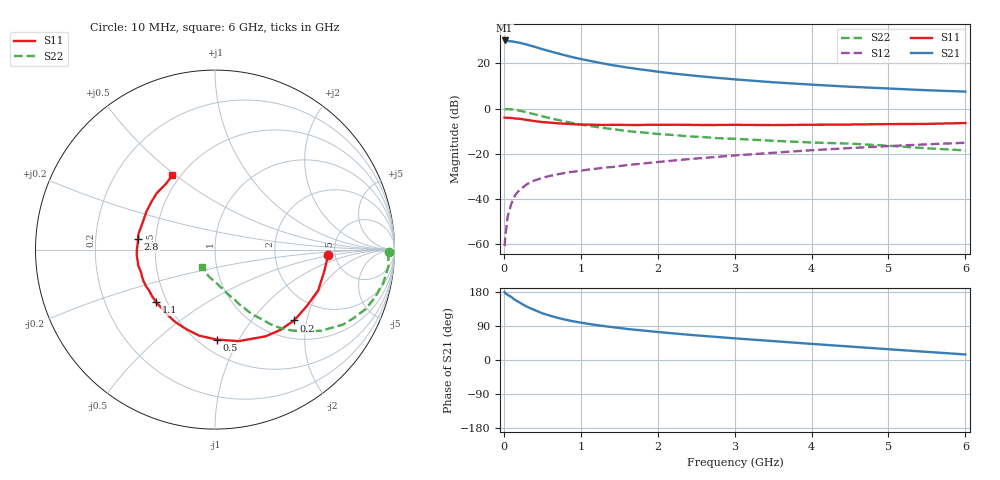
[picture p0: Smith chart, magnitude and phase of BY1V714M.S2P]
! SIEMENS Small Signal Semiconductors
! BFY420
! Si NPN RF SIEGET Grounded Emitter Transistor in MICRO-X
! VCE = 1.75 V  IC = 14 mA
! Common Emitter S-Parameters:  October  1996
# GHz  S  MA  R  50
!  f  S11  S21  S12  S22
! GHz  MAG  ANG  MAG  ANG  MAG  ANG  MAG  ANG
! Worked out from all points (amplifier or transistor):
!   36 points, 10 MHz to 6 GHz, reference 50 ohm
!   highest |S21| = 30.1 dB at 10 MHz (marker M1)
!   |S21| within 3 dB of that: start of sweep to 419.6 MHz
!   unconditionally stable (mu >= 1): 2.221 GHz to end of sweep
!   at 250 MHz: K = 0.23, MSG = 31.8 dB, |S12| = -34.8 dB
!   at 1.4 GHz: K = 0.84, MSG = 22.6 dB, |S12| = -25.9 dB
!   at 6 GHz: K = 1.09, MAG = 9.5 dB, |S12| = -15.2 dB
!   S11 on the Smith chart (normalised r, x): 10 MHz: 4.34, -0.42; 200 MHz: 1.39, -1.69; 500 MHz: 0.61, -0.81; 1.1 GHz: 0.44, -0.32; 2.8 GHz: 0.40, +0.06; 6 GHz: 0.45, +0.49
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0.01  0.6284 -2.7  32.05 179.1  0.0009 103.7  0.9694 -0.9
0.02  0.627 -4.9  32.02 176.2  0.0015 81.4  0.9658 -1.9
0.1  0.6183 -21.6  30.62 165.8  0.008 81.4  0.9558 -11.2
0.15  0.6003 -31.8  29.59 158.1  0.0124 76.6  0.93 -16.7
0.2  0.5919 -41.8  28.63 152.4  0.0155 73.6  0.9017 -21.6
0.25  0.5764 -51.1  27.32 146.1  0.0181 68.8  0.8616 -26.3
0.3  0.5591 -59.8  25.94 140.7  0.0212 65.9  0.8262 -30.4
0.4  0.5269 -75.4  23.24 131.8  0.0257 60.7  0.7451 -37.3
0.5  0.5016 -88.9  20.55 123.3  0.0292 57.6  0.6736 -42.8
0.6  0.4871 -100.7  18.46 117.0  0.0323 55.7  0.6127 -47.1
0.7  0.4708 -110.0  16.63 111.3  0.035 54.0  0.5601 -50.7
0.8  0.4605 -118.7  14.97 106.4  0.0377 52.6  0.5139 -53.6
0.9  0.45 -125.4  13.59 102.2  0.04 52.3  0.475 -55.6
1.1  0.4397 -138.4  11.53 95.3  0.0446 51.9  0.4162 -60.0
1.3  0.4323 -147.8  9.866 89.5  0.0491 51.8  0.3701 -62.9
1.6  0.4339 -159.7  8.092 82.0  0.0558 51.7  0.3191 -67.1
2.2  0.4373 -175.7  5.952 70.3  0.0705 50.6  0.2592 -73.7
2.8  0.433 172.0  4.725 60.3  0.0859 48.2  0.2197 -79.4
3.5  0.4303 159.3  3.809 49.9  0.1049 44.6  0.1934 -85.7
4.5  0.4425 143.5  3.031 35.5  0.1331 37.1  0.1671 -95.4
5.5  0.4568 126.9  2.537 21.5  0.1613 28.4  0.1318 -113.3
6  0.4775 119.8  2.366 14.6  0.1747 23.6  0.1185 -126.3
